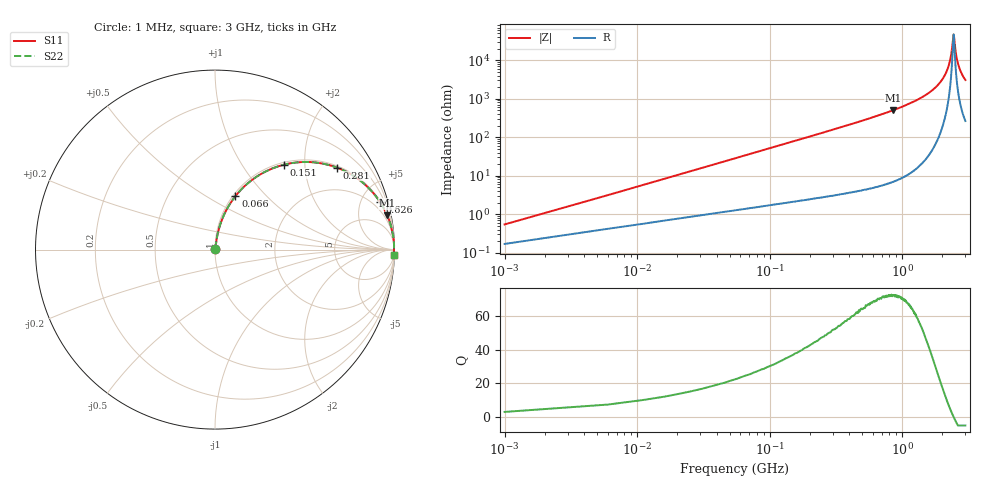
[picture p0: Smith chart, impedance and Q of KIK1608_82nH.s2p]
!version-2
!date-01.2022
!Series
# MHz S RI R 50
!Freq ReS11 ImS11 ReS21 ImS21 ReS12 ImS12 ReS22 ImS22
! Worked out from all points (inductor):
!   601 points, 1 MHz to 3 GHz, reference 50 ohm
!   read as one part in series: L = 82 nH near 16 MHz
!   highest Q = 72.3 at 851 MHz (marker M1), where L = 93.3 nH
!   self-resonance near 2.445 GHz
!   S11 on the Smith chart (normalised r, x): 1 MHz: 1.00, +0.01; 66 MHz: 1.03, +0.68; 151 MHz: 1.04, +1.56; 281 MHz: 1.06, +2.93; 626 MHz: 1.10, +6.90; 3 GHz: 6, -61
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1  0.00172 0.00513  0.9983 -0.00513  0.9983 -0.00513  0.00172 0.00513
21  0.019 0.1053  0.981 -0.1053  0.981 -0.1053  0.019 0.1053
26  0.0258 0.1294  0.9742 -0.1294  0.9742 -0.1294  0.0258 0.1294
41  0.0522 0.1981  0.9478 -0.1981  0.9478 -0.1981  0.0522 0.1981
66  0.1135 0.2976  0.8865 -0.2976  0.8865 -0.2976  0.1135 0.2976
151  0.3821 0.4726  0.6179 -0.4726  0.6179 -0.4726  0.3821 0.4726
281  0.6795 0.4568  0.3205 -0.4568  0.3205 -0.4568  0.6795 0.4568
501  0.8751 0.3229  0.1249 -0.3229  0.1249 -0.3229  0.8751 0.3229
626  0.9193 0.2652  0.0807 -0.2652  0.0807 -0.2652  0.9193 0.2652
851  0.9589 0.1917  0.0411 -0.1917  0.0411 -0.1917  0.9589 0.1917
1005  0.9728 0.1556  0.0272 -0.1556  0.0272 -0.1556  0.9728 0.1556
1505  0.992 0.0793  0.00804 -0.0793  0.00804 -0.0793  0.992 0.0793
2005  0.9972 0.0316  0.00279 -0.0316  0.00279 -0.0316  0.9972 0.0316
2165  0.9977 0.0193  0.00227 -0.0193  0.00227 -0.0193  0.9977 0.0193
2280  0.9979 0.0111  0.00211 -0.0111  0.00211 -0.0111  0.9979 0.0111
2355  0.9979 0.00599  0.00209 -0.00599  0.00209 -0.00599  0.9979 0.00599
2440  0.9979 0.000393  0.00213 -0.000393  0.00213 -0.000393  0.9979 0.000393
2460  0.9979 -0.000895  0.00215 0.000895  0.00215 0.000895  0.9979 -0.000895
2505  0.9978 -0.00376  0.00221 0.00376  0.00221 0.00376  0.9978 -0.00376
2575  0.9977 -0.00811  0.00234 0.00811  0.00234 0.00811  0.9977 -0.00811
2675  0.9974 -0.0141  0.00258 0.0141  0.00258 0.0141  0.9974 -0.0141
3000  0.9961 -0.0323  0.00385 0.0323  0.00385 0.0323  0.9961 -0.0323
